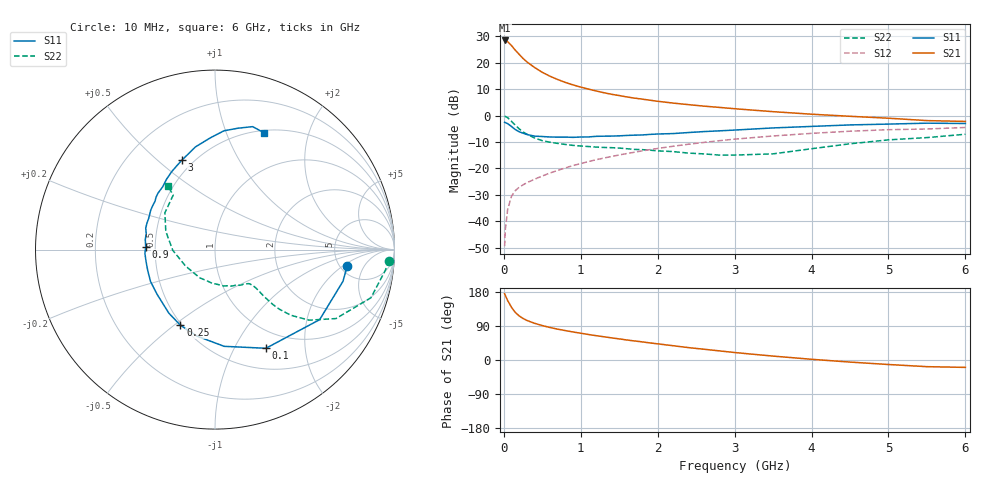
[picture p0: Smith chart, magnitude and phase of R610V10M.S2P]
! SIEMENS Small Signal Semiconductors
! BFR193
! Si NPN RF Bipolar Junction Transistor in SOT23
! VCE = 10 V  IC = 10 mA
! Common Emitter S-Parameters:  May  1996
# GHz  S  MA  R  50
!  f  S11  S21  S12  S22
! GHz  MAG  ANG  MAG  ANG  MAG  ANG  MAG  ANG
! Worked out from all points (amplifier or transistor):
!   36 points, 10 MHz to 6 GHz, reference 50 ohm
!   highest |S21| = 28.4 dB at 10 MHz (marker M1)
!   |S21| within 3 dB of that: start of sweep to 129.9 MHz
!   unconditionally stable (mu >= 1): 765 MHz to 2.07 GHz
!   at 250 MHz: K = 0.62, MSG = 23.9 dB, |S12| = -26.2 dB
!   at 1.4 GHz: K = 1.04, MAG = 10.5 dB, |S12| = -15.5 dB
!   at 6 GHz: K = 0.94, MSG = 1.1 dB, |S12| = -4.5 dB
!   S11 on the Smith chart (normalised r, x): 10 MHz: 5.83, -2.32; 100 MHz: 0.76, -1.35; 250 MHz: 0.49, -0.53; 900 MHz: 0.44, +0.02; 3 GHz: 0.43, +0.60; 6 GHz: 0.53, +1.37
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0.01  0.7429 -6.9  26.16 175.0  0.0034 82.0  0.9726 -3.6
0.02  0.7346 -13.9  25.86 170.0  0.0071 80.0  0.9551 -7.1
0.05  0.7016 -33.8  24.73 156.8  0.017 73.5  0.909 -17.2
0.1  0.6187 -62.7  20.88 138.8  0.0299 63.9  0.7756 -29.7
0.15  0.5413 -84.6  17.09 125.3  0.0382 58.0  0.6548 -36.9
0.2  0.4925 -101.7  14.27 116.2  0.0442 56.3  0.5584 -40.9
0.25  0.4633 -114.6  11.94 109.6  0.049 55.5  0.4888 -42.8
0.3  0.4376 -126.0  10.29 104.4  0.0538 56.2  0.4432 -43.5
0.4  0.4075 -142.4  8.065 96.8  0.0626 57.3  0.3758 -43.7
0.5  0.4009 -153.5  6.533 90.8  0.072 59.1  0.3345 -43.3
0.6  0.3927 -162.4  5.519 85.8  0.0819 60.1  0.3126 -43.2
0.7  0.3898 -170.1  4.782 81.4  0.0918 61.3  0.2972 -43.4
0.9  0.3865 177.6  3.782 73.9  0.1133 62.3  0.2724 -44.5
1.1  0.3935 166.9  3.153 67.3  0.1348 62.6  0.2593 -47.4
1.3  0.4068 158.8  2.695 61.3  0.1571 61.7  0.249 -50.7
1.6  0.4202 148.5  2.239 52.8  0.191 60.0  0.2357 -57.6
2.2  0.4556 129.7  1.716 37.7  0.2625 54.5  0.2082 -76.8
3  0.5308 110.4  1.343 19.7  0.3576 44.4  0.1788 -118.2
3.5  0.5823 100.8  1.181 10.3  0.4102 37.0  0.1886 -151.6
4.5  0.6638 85.7  0.966 -5.5  0.5051 22.5  0.2922 159.7
5.5  0.7164 73.0  0.801 -17.6  0.5559 7.2  0.3825 127.5
6  0.7062 67.3  0.773 -19.5  0.5942 2.7  0.4424 126.5
